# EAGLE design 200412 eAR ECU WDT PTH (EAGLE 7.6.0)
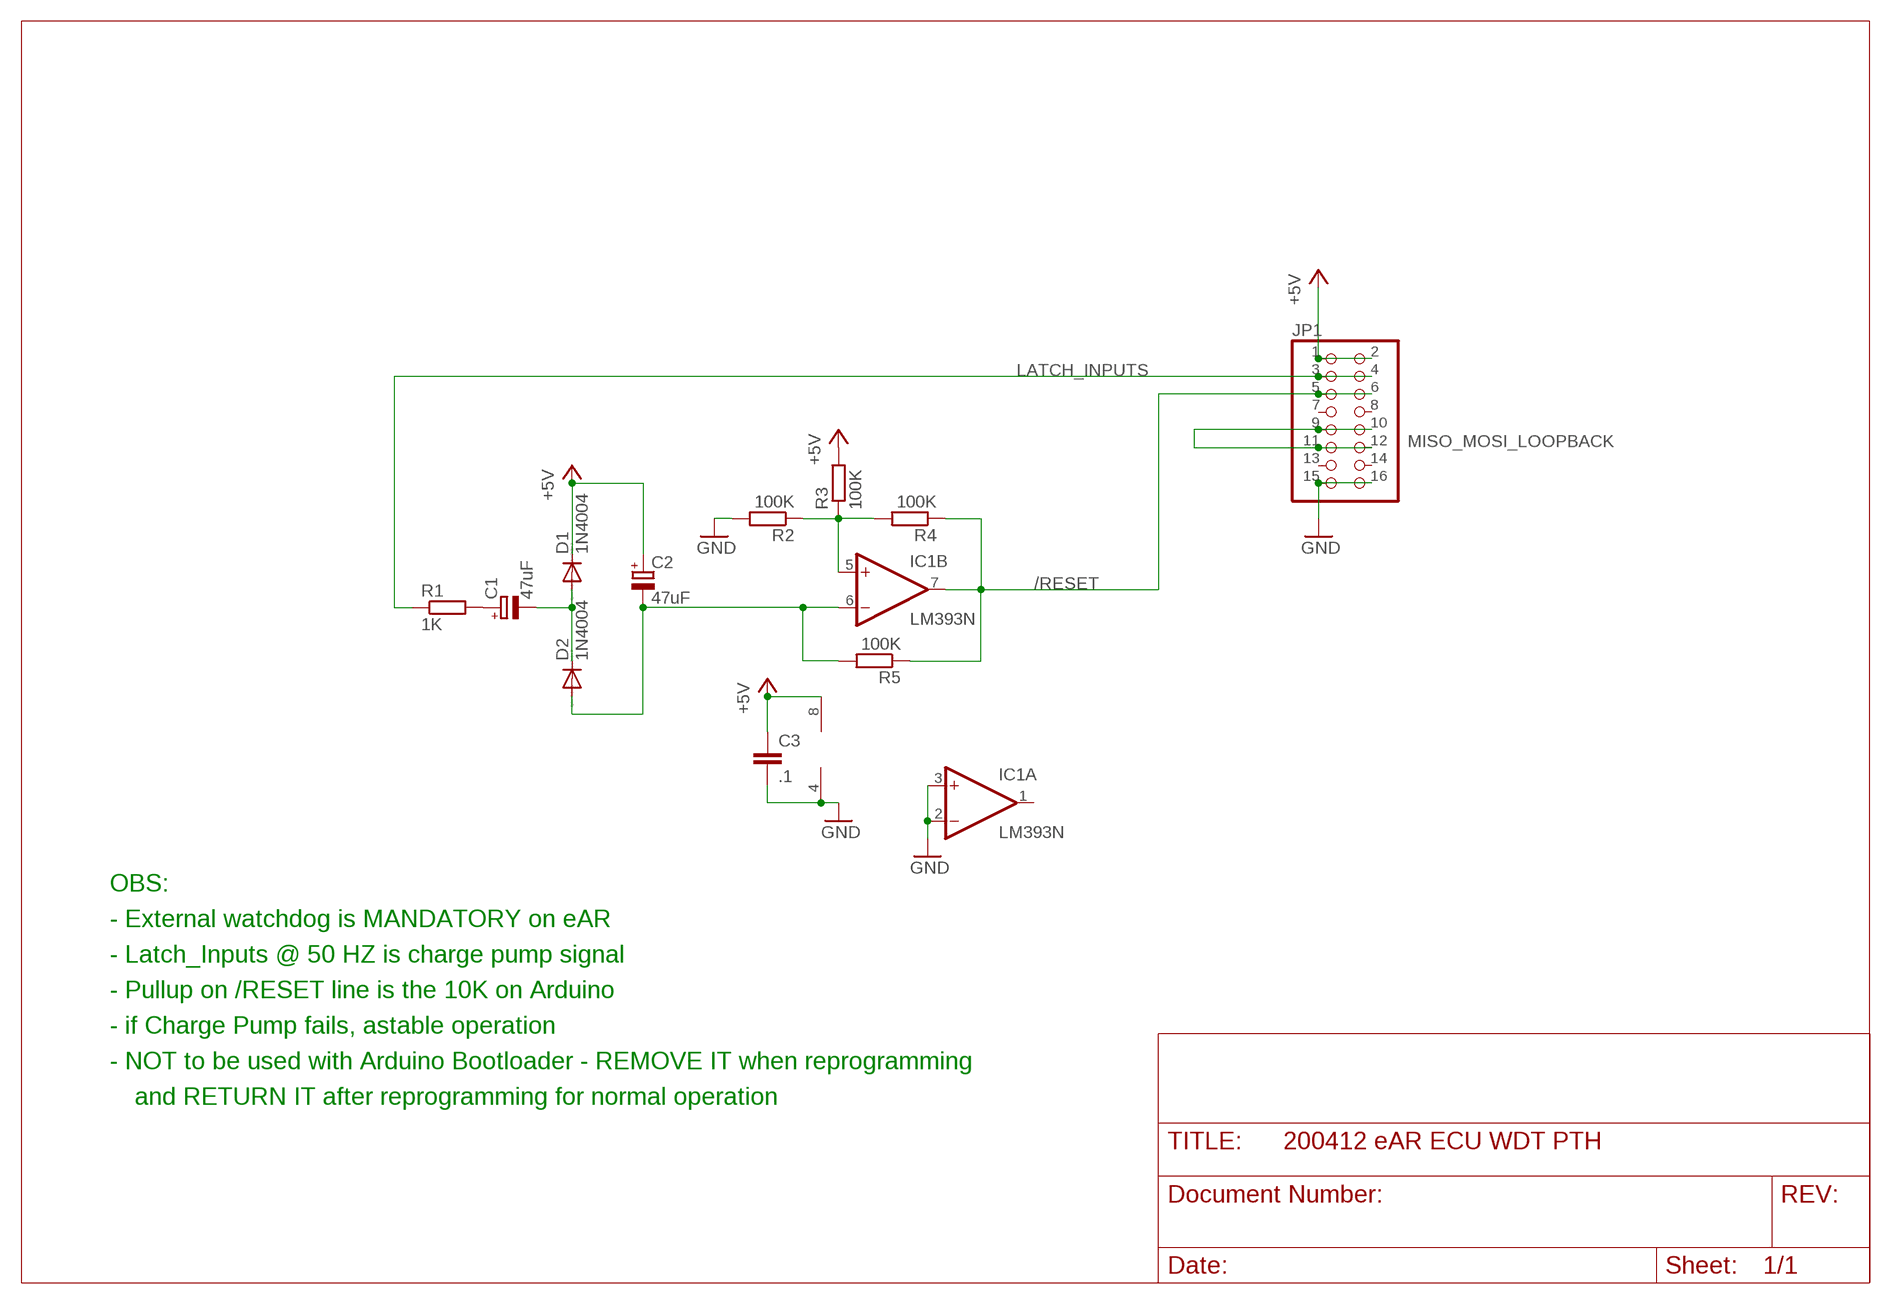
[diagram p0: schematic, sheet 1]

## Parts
C1  47uF  CPOL-EUE2.5-5  [E2,5-5]
C2  47uF  CPOL-EUE2.5-5  [E2,5-5]
C3  .1  C-EU050-025X075  [C050-025X075]
D1  1N4004  [DO41-10]
D2  1N4004  [DO41-10]
IC1  LM393N  [DIL08]
JP1  PINHD-2X8  [2X08]
R1  1K  R-EU_0207/10  [0207/10]
R2  100K  R-EU_0207/10  [0207/10]
R3  100K  R-EU_0207/10  [0207/10]
R4  100K  R-EU_0207/10  [0207/10]
R5  100K  R-EU_0207/10  [0207/10]

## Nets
+5V: C2.+ C3.1 D1.C IC1.8(P:V+) JP1.1 JP1.2 R3.2
/RESET: IC1.7(B:OUT) JP1.5 JP1.6 R4.1 R5.1
GND: C3.2 IC1.2(A:-IN) IC1.3(A:+IN) IC1.4(P:V-) JP1.15 JP1.16 R2.2
LATCH_INPUTS: JP1.3 JP1.4 R1.1
MISO_MOSI_LOOPBACK: JP1.9 JP1.10 JP1.11 JP1.12
N$1: C1.+ R1.2
N$3: C2.- D2.A IC1.6(B:-IN) R5.2
N$4: IC1.5(B:+IN) R2.1 R3.1 R4.2
N$5: C1.- D1.A D2.C
Unconnected: IC1.1(A:OUT) JP1.7 JP1.8 JP1.13 JP1.14

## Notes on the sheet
- OBS:
- - External watchdog is MANDATORY on eAR
- - Latch_Inputs @ 50 HZ is charge pump signal
- - Pullup on /RESET line is the 10K on Arduino
- - if Charge Pump fails, astable operation
- - NOT to be used with Arduino Bootloader - REMOVE IT when reprogramming
- and RETURN IT after reprogramming for normal operation

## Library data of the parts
C1 C2 = rcl:CPOL-EU: POLARIZED CAPACITOR, European symbol
C3 = rcl:C-EU: CAPACITOR, European symbol
D1 D2 = diode:1N4004: DIODE
IC1 = linear:LM393: COMPARATOR
JP1 = pinhead:PINHD-2X8: PIN HEADER
R1-R5 = rcl:R-EU_: RESISTOR, European symbol

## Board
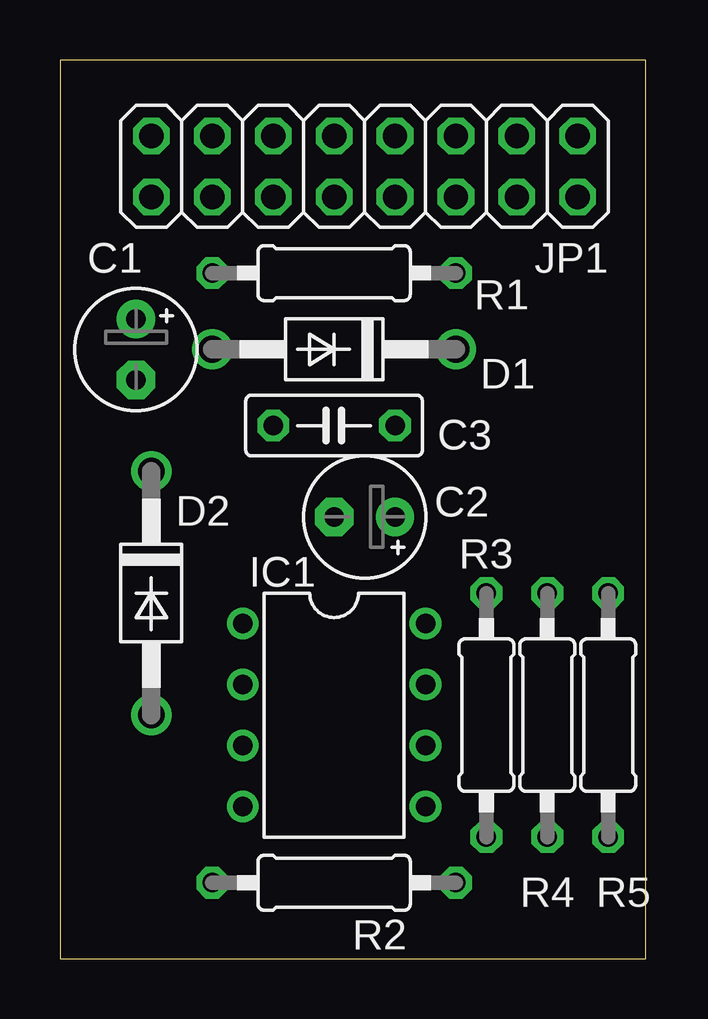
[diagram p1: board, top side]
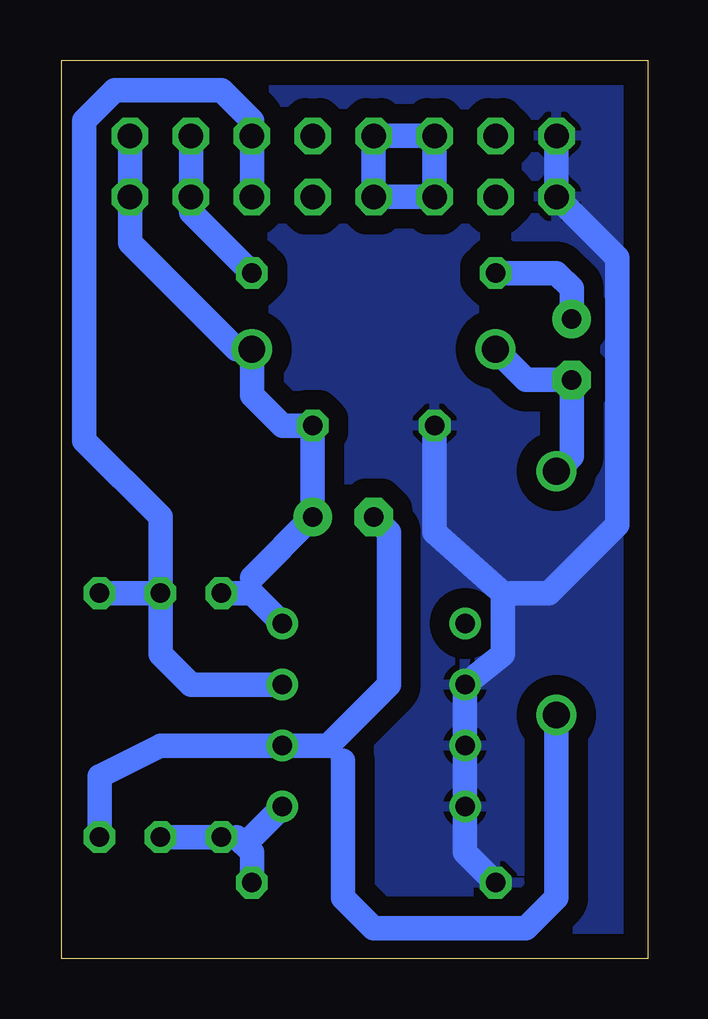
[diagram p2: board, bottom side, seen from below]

Size 24.43 x 37.45 mm. Coordinates in mm from the lower left corner, seen from the top.
Outline: 0,0 24.43,0 24.43,37.45 0,37.45 0,0
Copper layers (1*16): Top 0.035mm / dielectric 1.5mm / Bottom 0.035mm
Design rules "default": minimum track width 10mil, minimum drill 24mil, track to track 8mil, track to pad 8mil, pad to pad 8mil, via to via 8mil, smd to smd 8mil, copper to edge 40mil, drill to drill 8mil, minimum pad ring 10mil, minimum via ring 8mil, stop-mask expansion 4mil, vias tented up to drill 0mil, thermal gap 10mil

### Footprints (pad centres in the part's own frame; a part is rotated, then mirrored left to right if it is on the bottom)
E2,5-5 = drill 0.813 pad 1.6: + -1.27,0 | drill 0.813 pad 1.6 octagon: - 1.27,0
C050-025X075 = drill 0.813 octagon: 1 -2.54,0; 2 2.54,0
DO41-10 = drill 1.118: A 5.08,0; C -5.08,0
DIL08 = drill 0.813 pad 1.27: 1 -3.81,-3.81; 2 -1.27,-3.81; 3 1.27,-3.81; 4 3.81,-3.81; 5 3.81,3.81; 6 1.27,3.81; 7 -1.27,3.81; 8 -3.81,3.81
2X08 = drill 1.016 octagon: 1 -8.89,-1.27; 2 -8.89,1.27; 3 -6.35,-1.27; 4 -6.35,1.27; 5 -3.81,-1.27; 6 -3.81,1.27; 7 -1.27,-1.27; 8 -1.27,1.27; 9 1.27,-1.27; 10 1.27,1.27; 11 3.81,-1.27; 12 3.81,1.27; 13 6.35,-1.27; 14 6.35,1.27; 15 8.89,-1.27; 16 8.89,1.27
0207/10 = drill 0.813 octagon: 1 -5.08,0; 2 5.08,0

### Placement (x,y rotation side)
C1  3.17,25.4 270 top
C2  12.7,18.41 180 top
C3  11.43,22.23 180 top
D1  11.43,25.4 180 top
D2  3.81,15.24 270 top
IC1  11.43,10.16 270 top
JP1  12.7,33.02 180 top
R1  11.43,28.57 180 top
R2  11.43,3.17 180 top
R3  17.78,10.16 90 top
R4  20.32,10.16 270 top
R5  22.86,10.16 270 top

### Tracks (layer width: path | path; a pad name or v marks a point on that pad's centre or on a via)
+5V
  Bottom 0.61: 16.51,15.24 16.51,15.88 | D1.C 17.14,25.4
  Bottom 1.016: R3.2 16.51,15.24 IC1.8 | JP1.1 JP1.2 21.59,29.84 17.14,25.4 | 16.51,15.88 C2.+ C3.1 15.24,22.23 16.51,23.5 D1.C
/RESET
  Bottom 0.61: 16.51,34.92 JP1.5
  Bottom 1.016: IC1.7 19.05,11.43 20.32,12.7 R4.1 | R5.1 R4.1 | JP1.6 JP1.5 | R4.1 20.32,18.41 23.5,21.59 23.5,34.92 22.23,36.2 17.78,36.2 16.51,34.92
GND
  Bottom 1.016: 6.03,14.92 6.03,12.7 IC1.2 IC1.3 IC1.4 7.62,4.45 R2.2 | 6.03,14.92 6.03,15.24 8.89,17.78 C3.2 | JP1.15 JP1.16 1.27,29.21 1.27,18.1 4.13,15.24 5.71,15.24 6.03,14.92
  pour Bottom (isolate 0.813): 0,37.47 24.13,37.47 24.13,0 0,0
LATCH_INPUTS
  Bottom 0.61: 19.05,31.11 JP1.4
  Bottom 1.016: JP1.4 JP1.3 | R1.1 19.05,31.11
MISO_MOSI_LOOPBACK
  Bottom 1.016: JP1.11 JP1.9 JP1.10 JP1.12 JP1.11
N$1
  Bottom 1.016: C1.+ 3.17,27.94 3.81,28.57 R1.2
N$3
  Bottom 0.61: 12.7,8.26 13.34,8.89
  Bottom 1.016: R5.2 22.86,7.62 20.32,8.89 IC1.6 13.34,8.89 10.79,11.43 10.79,17.78 C2.- | D2.A 3.81,2.54 5.08,1.27 11.43,1.27 12.7,2.54 12.7,8.26
N$4
  Bottom 0.61: 16.51,5.08 17.14,5.08 R3.1
  Bottom 1.016: R4.2 R3.1 | IC1.5 16.51,5.08 | R2.1 16.51,4.45 17.14,5.08
N$5
  Bottom 1.016: D1.A 5.08,24.13 C1.- 3.17,20.95 D2.C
